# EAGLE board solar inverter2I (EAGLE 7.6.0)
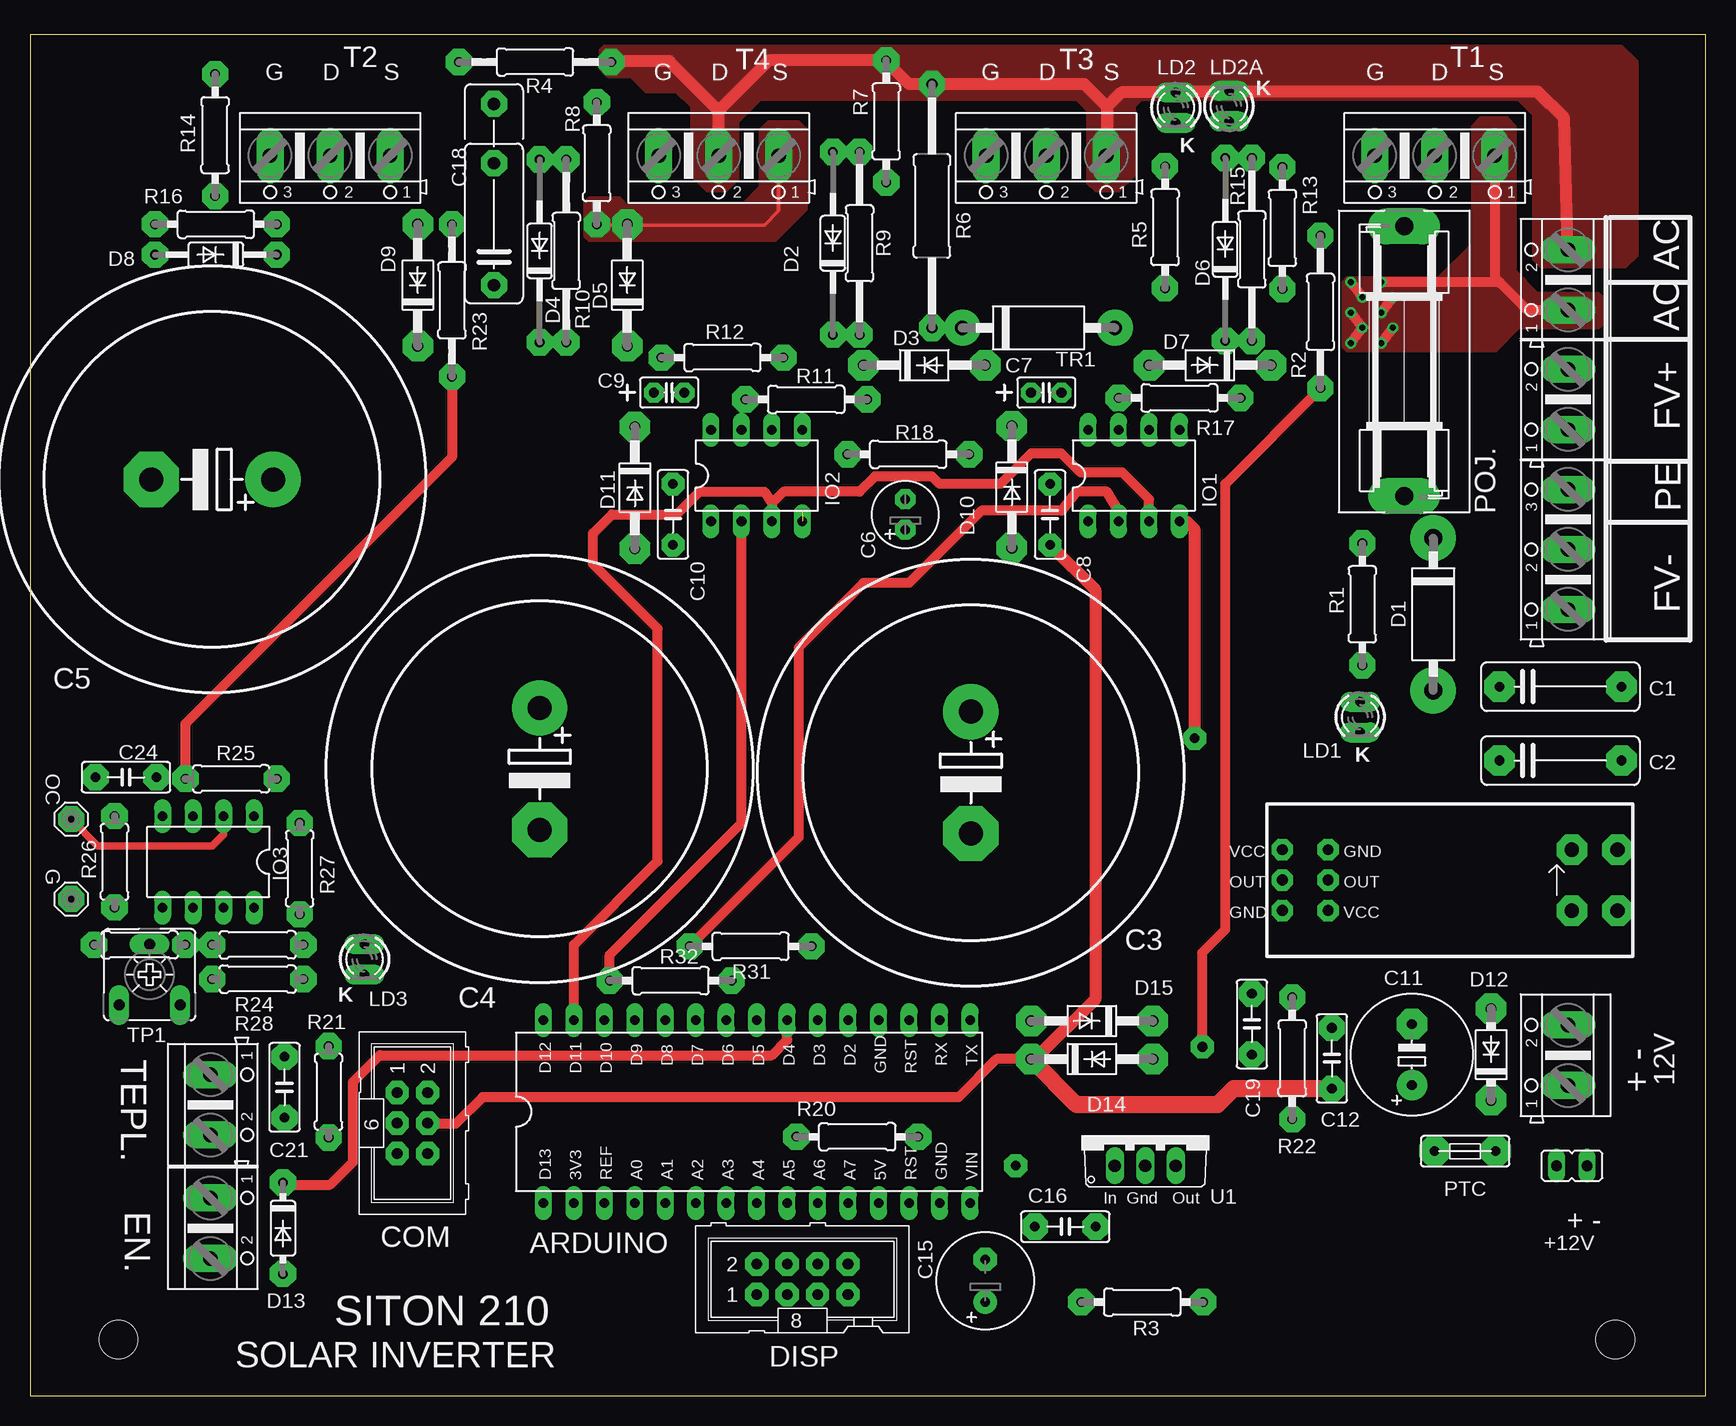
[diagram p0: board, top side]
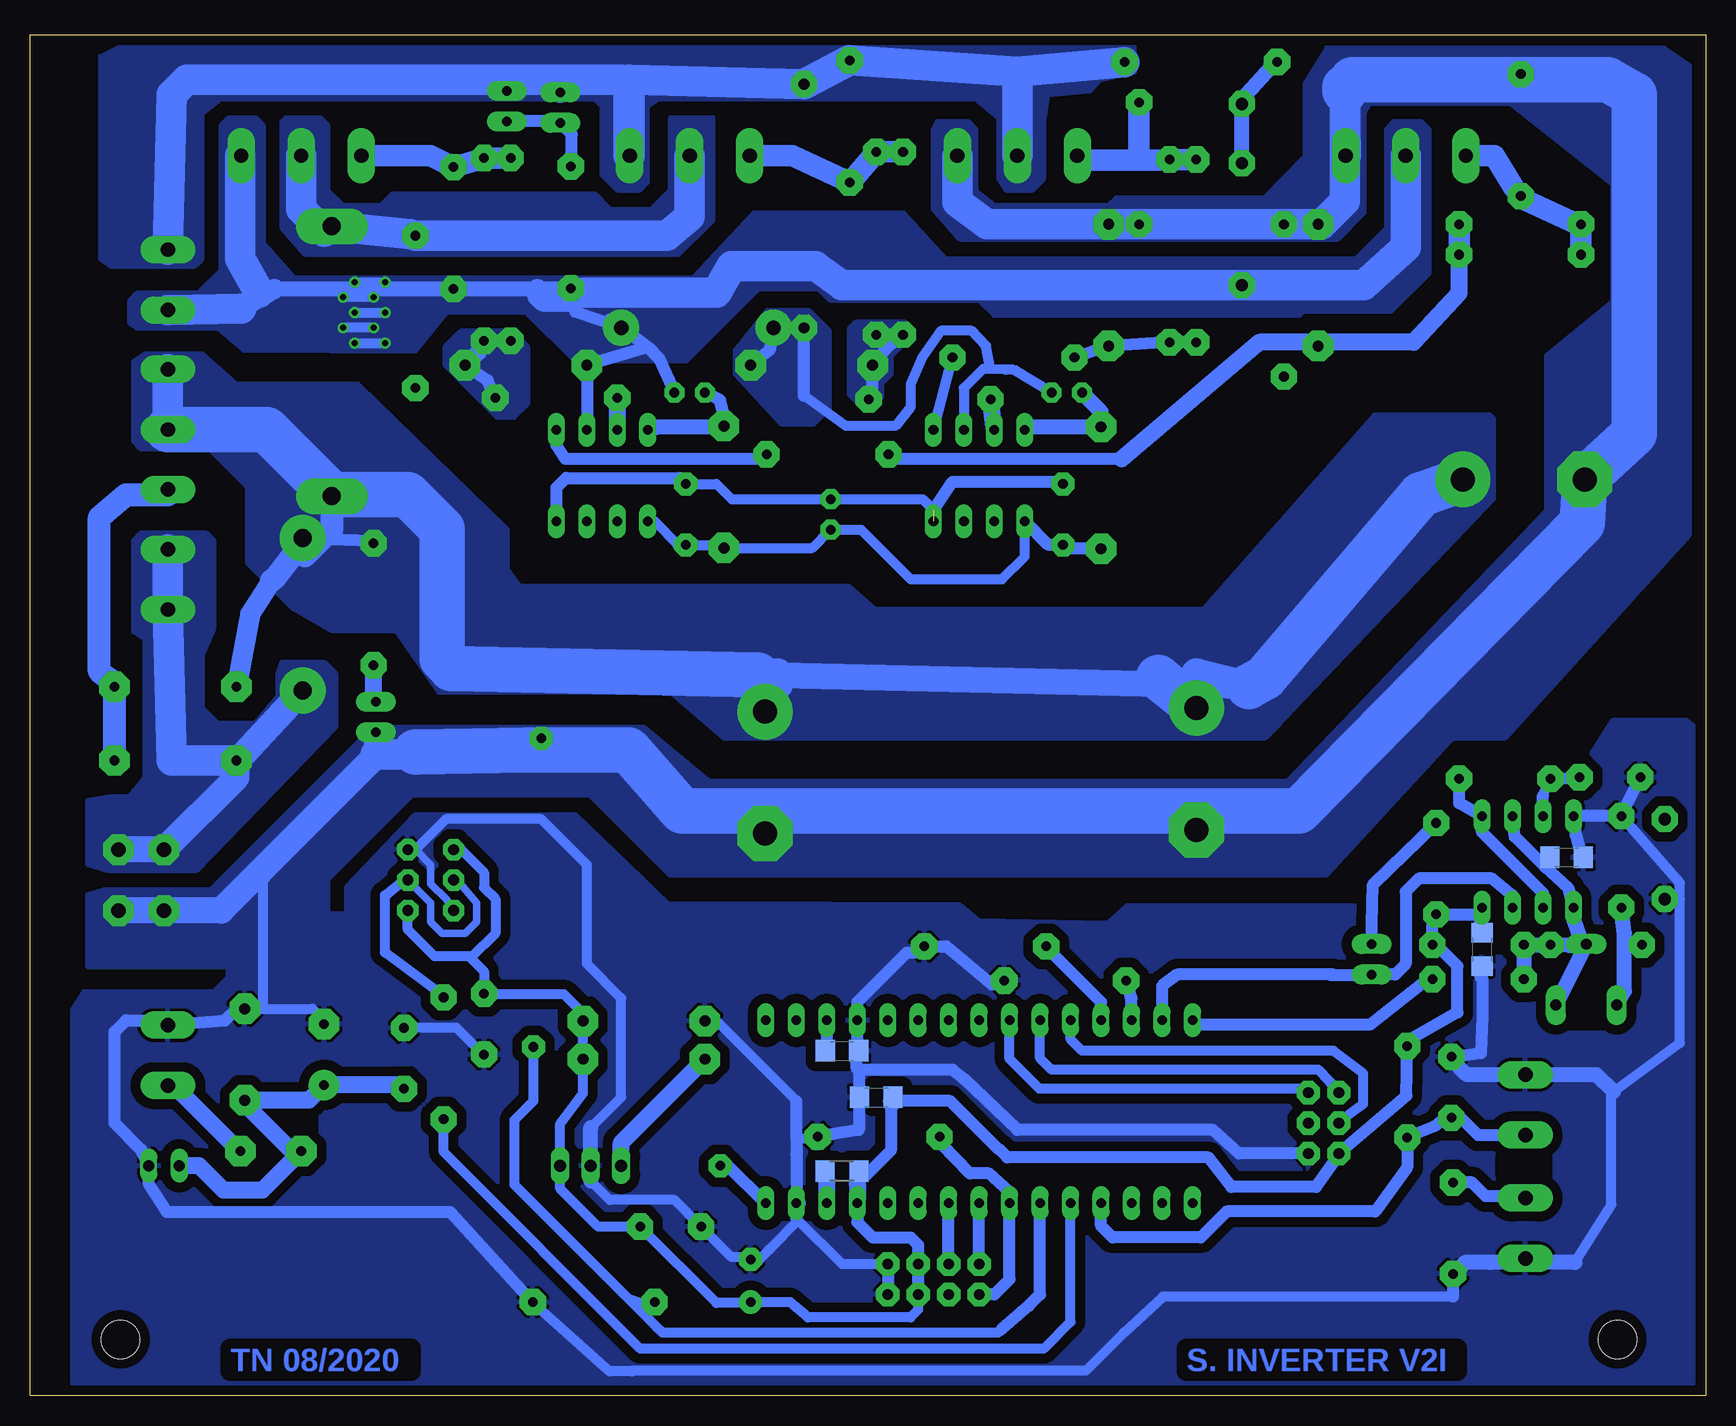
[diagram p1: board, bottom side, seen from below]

Size 139.7 x 113.47 mm. Coordinates in mm from the lower left corner, seen from the top.
Outline: 139.7,113.47 0,113.47 0,0 139.7,0 139.7,113.47
Copper layers (1*16): Top 0.035mm / dielectric 1.5mm / Bottom 0.035mm
Design rules "default *": minimum track width 10mil, minimum drill 24mil, track to track 8mil, track to pad 8mil, pad to pad 8mil, via to via 8mil, smd to smd 8mil, copper to edge 15mil, drill to drill 8mil, minimum pad ring 10mil, minimum via ring 8mil, stop-mask expansion 4mil, vias tented up to drill 0mil, thermal gap 10mil
Holes 3.2 mm at 132.14,4.7 7.37,4.7
bRestrict: area 71.6,27.9 to 72.3,30.2; area 68.9,24.1 to 69.5,25.8; area 74.3,15.4 to 77,16.5; area 7.6,31.2 to 12.3,37.3; area 13.6,18.5 to 16.8,19.8; area 116.5,22 to 118.4,23.6

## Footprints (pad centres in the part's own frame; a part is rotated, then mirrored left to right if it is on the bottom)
AK500/2 = drill 1.2 pad 2.311 long: 1 -2.515,0; 2 2.515,0
JP1 = drill 0.9 pad 1.422 long: 1 0,-1.27; 2 0,1.27
DIL30 = drill 0.8 pad 1.422 long: 1 -16.51,-7.62; 2 -13.97,-7.62; 3 -11.43,-7.62; 4 -8.89,-7.62; 5 -6.35,-7.62; 6 -3.81,-7.62; 7 -1.27,-7.62; 8 1.27,-7.62; 9 3.81,-7.62; 10 6.35,-7.62; 11 8.89,-7.62; 12 11.43,-7.62; 13 13.97,-7.62; 14 16.51,-7.62; 15 19.05,-7.62; 18 19.05,7.62; 19 16.51,7.62; 20 13.97,7.62; 21 11.43,7.62; 22 8.89,7.62; 23 6.35,7.62; 24 3.81,7.62; 25 1.27,7.62; 26 -1.27,7.62; 27 -3.81,7.62; 28 -6.35,7.62; 29 -8.89,7.62; 30 -11.43,7.62; 31 -13.97,7.62; 32 -16.51,7.62
C10B4 = drill 0.8 pad 2.54 octagon: 1 -5.08,0; 2 5.08,0
EB35D = drill 2 pad 4.597: + -5.08,0 | drill 2 pad 4.597 octagon: - 5.08,0
E2,5-6 = drill 0.8 pad 1.676 octagon: + -1.27,0; - 1.27,0
C025-025X050+ = drill 0.8 pad 1.676 octagon: 1 -1.27,0; 2 1.27,0
C050-025X075 = drill 0.8 pad 1.93 octagon: 1 -2.54,0; 2 2.54,0
E5-10,5 = drill 0.8 pad 2.54: + -2.54,0 | drill 0.8 pad 2.54 octagon: - 2.54,0
C050-025X075' = drill 0.8 pad 2.184 octagon: 1 -2.54,0; 2 2.54,0
C1206 = smd 1.6 x 1.8: 1 -1.4,0; 2 1.4,0
E3,5-8 = drill 0.8 pad 1.93: + -1.778,0 | drill 0.8 pad 1.93 octagon: - 1.778,0
C10-15B6 = drill 1.016 pad 2.159 octagon: 1 -5.08,0; 2 5.08,0; 3 10.033,0
ML6 = drill 0.9 pad 1.93 octagon: 1 -2.54,-1.27; 2 -2.54,1.27; 3 0,-1.27; 4 0,1.27; 5 2.54,-1.27; 6 2.54,1.27
DO15-12-1.5 = drill 1.5 pad 3.81: A 6.35,0; C -6.35,0
DO35-15 = drill 0.8 pad 2.184 octagon: A 7.62,0; C -7.62,0
DO41-10 = drill 0.9 pad 2.54 octagon: A 5.08,0; C -5.08,0
DO35-10 = drill 0.8 pad 2.184 octagon: A 5.08,0; C -5.08,0
DO41-7 = drill 0.9 pad 2.54 octagon: A 3.81,0; C -3.81,0
DO35-7 = drill 0.8 pad 2.184 octagon: A 3.81,0; C -3.81,0
ML8 = drill 0.9 pad 1.93 octagon: 1 -5.08,-1.27; 2 -5.08,1.27; 3 -2.54,-1.27; 4 -2.54,1.27; 5 0,-1.27; 6 0,1.27; 7 2.54,-1.27; 8 2.54,1.27
ACS712V2 = drill 0.9 pad 1.778 octagon: P$1 3.81,5.08; P$2 0,0; P$3 0,2.54; P$4 0,5.08; P$5 3.81,2.54; P$7 3.81,0 | drill 1.2 pad 2.54 octagon: P$6 24.13,0; P$8 24.13,5.08; P$9 27.94,5.08; P$10 27.94,0
AK500/3 = drill 1.2 pad 2.311 long: 1 -5.004,0; 2 0,0; 3 5.004,0
MCS10B = drill 1.016 pad 2.159 octagon: MP 0,0
DIL08 = drill 0.8 pad 1.422 long: 1 -3.81,-3.81; 2 -1.27,-3.81; 3 1.27,-3.81; 4 3.81,-3.81; 5 3.81,3.81; 6 1.27,3.81; 7 -1.27,3.81; 8 -3.81,3.81
LED3MM = drill 0.8 pad 1.676 long: A -1.27,0; K 1.27,0
POJISTKA = drill 1.5 pad 3 long: 1 -11.252,0; 2 11.252,0
PTC_FUSE = drill 0.8 pad 2.54 octagon: 1 -2.54,0; 2 2.54,0
0207/10 = drill 0.8 pad 2.184 octagon: 1 -5.08,0; 2 5.08,0
0207/12 = drill 0.8 pad 2.184 octagon: 1 -6.35,0; 2 6.35,0
0309/20 = drill 0.9 pad 2.184 octagon: 1 -10.16,0; 2 10.16,0
0207/15 = drill 0.8 pad 2.184 octagon: 1 -7.62,0; 2 7.62,0
R1206 = smd 1.6 x 1.803: 1 -1.422,0; 2 1.422,0
0207/7 = drill 0.8 pad 2.184 octagon: 1 -3.81,0; 2 3.81,0
CA6V = drill 0.9 pad 1.676 long: A -2.54,-2.54; E 2.54,-2.54; S 0,2.54
DO15-12 = drill 1.2 pad 3: A 6.35,0; C -6.35,0
TO220V = drill 1.016 long: 1 -2.54,-2.54; 2 0,-2.54; 3 2.54,-2.54

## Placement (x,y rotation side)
12V  + 12V -  [AK500/2]  128.21,28.38 90 top
+12V  +12V-  [JP1]  128.52,19.18 90 top
ARDUINO  Arduino Nano  [DIL30]  59.31,23.69 0 top
C1  100n/275V  [C10B4]  127.57,59.12 0 top
C2  100n/275V  [C10B4]  127.57,52.96 0 top
C3  470u/450V  [EB35D]  78.42,51.94 270 top
C4  470u/450V  [EB35D]  42.48,52.26 270 top
C5  470u/450V  [EB35D]  15.18,76.39 180 top
C6  10u  [E2,5-6]  72.96,73.47 90 top
C7  10u  [C025-025X050+]  84.71,83.63 0 top
C8  100n  [C050-025X075]  85.03,73.47 270 top
C9  10u  [C025-025X050+]  53.28,83.63 0 top
C10  100n  [C050-025X075]  53.59,73.47 270 top
C11  470uF  [E5-10,5]  115.19,28.45 90 top
C12  100n  [C050-025X075']  108.52,28.13 90 top
C13  100n  [C1206]  69.15,24.89 0 bottom
C14  100n  [C1206]  72.01,28.77 0 bottom
C15  220uF  [E3,5-8]  79.63,9.59 90 top
C16  100n  [C050-025X075']  86.3,14.1 0 top
C18  15n  [C10-15B6]  38.67,97.66 90 top
C19  100n  [C050-025X075']  101.85,30.99 90 top
C21  100n  [C050-025X075']  21.21,25.72 270 top
C24  33n  [C050-025X075']  8,51.56 180 top
C25  100n  [C1206]  11.62,44.89 0 bottom
C26  100n  [C1206]  18.67,37.21 270 bottom
COM  [ML6]  31.88,22.73 270 top
D1  15A10G  [DO15-12-1.5]  116.97,65.15 270 top
D2  1N4148  [DO35-15]  66.93,96.08 90 top
D3  P6KE18A  [DO41-10]  74.55,85.92 0 top
D4  1N4148  [DO35-15]  42.48,95.44 90 top
D5  P6KE18A  [DO41-10]  49.78,92.58 90 top
D6  1N4148  [DO35-15]  99.63,95.57 90 top
D7  P6KE18A  [DO41-10]  98.36,85.92 180 top
D8  1N4148  [DO35-10]  15.49,95.12 180 top
D9  P6KE18A  [DO41-10]  32.32,92.58 90 top
D10  UF4007  [DO41-10]  81.85,75.76 270 top
D11  UF4007  [DO41-10]  50.42,75.69 270 top
D12  P6KE15A  [DO41-7]  121.79,28.45 90 top
D13  ZD5V1  [DO35-7]  21.08,13.97 270 top
D14  1N4007  [DO41-10]  88.52,28.07 0 top
D15  ZD5V6  [DO41-10]  88.52,31.24 180 top
DISP  [ML8]  65.66,9.72 0 top
E$2  [ACS712V2]  104.39,40.45 0 top
E$11  [AK500/3]  128.21,70.55 90 top
E$13  [AK500/2]  128.21,83.06 90 top
E$14  [AK500/2]  128.21,93.03 90 top
EN.  EN.  [AK500/2]  15.05,13.97 270 top
G  [MCS10B]  3.43,41.4 0 top
IO1  IR2104  [DIL08]  92.01,76.71 0 top
IO2  IR2104  [DIL08]  60.58,76.71 0 top
IO3  [DIL08]  14.86,44.51 180 top
LD1  [LED3MM]  110.87,56.58 270 top
LD2  [LED3MM]  95.5,107.38 270 top
LD2A  [LED3MM]  99.95,107.51 90 top
LD3  [LED3MM]  27.88,36.39 270 top
OC  [MCS10B]  3.43,48.07 0 top
POJ.  [POJISTKA]  114.55,86.23 90 top
PTC  400mA  [PTC_FUSE]  119.63,20.38 180 top
R1  300k  [0207/10]  111.06,65.98 90 top
R2  470K  [0207/12]  107.57,90.36 90 top
R3  5k6  [0207/10]  92.71,7.81 180 top
R4  10R  [0207/12]  42.1,111.19 0 top
R5  300k  [0207/10]  94.61,97.41 90 top
R6  0R1  [0309/20]  75.18,99.19 90 top
R7  22k  [0207/10]  71.37,106.24 90 top
R8  22k  [0207/10]  47.24,102.74 90 top
R9  100R  [0207/15]  69.15,96.08 90 top
R10  100R  [0207/15]  44.7,95.44 90 top
R11  10R  [0207/10]  64.71,83.06 180 top
R12  10R  [0207/10]  57.72,86.55 0 top
R13  22k  [0207/10]  104.39,97.35 90 top
R14  22k  [0207/10]  15.43,105.09 270 top
R15  100R  [0207/15]  101.85,95.57 90 top
R16  100R  [0207/10]  15.49,97.66 0 top
R17  10R  [0207/10]  95.82,83.19 180 top
R18  10R  [0207/10]  73.22,78.49 0 top
R19  1k  [R1206]  72.01,18.73 0 bottom
R20  10k  [0207/10]  68.96,21.59 0 top
R21  2k2  [0207/7]  24.89,25.34 90 top
R22  560  [0207/10]  105.22,28.13 90 top
R23  10k  [0207/12]  35.18,91.31 90 top
R24  100k  [0207/7]  18.99,37.59 0 top
R25  33k  [0207/7]  16.76,51.44 0 top
R26  1k5  [0207/7]  7.05,44.51 90 top
R27  1k  [0207/7]  22.48,43.94 90 top
R28  560  [0207/7]  18.99,34.73 0 top
R31  10k  [0207/10]  60.07,37.47 0 top
R32  10k  [0207/10]  53.4,34.61 0 top
T1  47N60  [AK500/3]  117.09,103.38 180 top
T2  47N60  [AK500/3]  25.02,103.38 180 top
T3  47N60  [AK500/3]  84.71,103.38 180 top
T4  47N60  [AK500/3]  57.4,103.38 180 top
TEPL.  TEPL.  [AK500/2]  15.05,24.26 270 top
TP1  5k  [CA6V]  9.97,35.12 0 top
TP2  [0207/7]  9.14,37.59 180 top
TR1  1,5KE440CA  [DO15-12]  84.07,89.03 0 top
U1  LM7805  [TO220V]  92.96,21.72 0 top

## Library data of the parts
12V +12V ARDUINO C1-C6 C12-C14 C16 C18 C19 C21 C24-C26 COM D1-D15 DISP E$2 E$11 E$13 E$14 EN. IO1-IO3 POJ. PTC R1-R28 R31 R32 T1-T4 TEPL. TP1 TP2 TR1 = 11moje
C7-C11 C15 = 12moje
G OC = solpad
LD1 LD2 LD2A LD3 = 10moje
U1 = linear

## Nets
+5V: ARDUINO.12 C13.2 C15.+ C16.2 C19.2 C26.1 COM.5 D14.A D15.C DISP.5 DISP.6 E$2.P$4 E$2.P$7 IO3.8 R19.2 R21.2 R24.2 R27.1 U1.3
+12V: +12V.2 C6.+ C8.2 C10.2 C11.+ C12.1 COM.4 D10.A D11.A D12.C D14.C IO1.1 IO2.1 PTC.2 U1.1
AC1: E$14.2 LD2.A LD2A.K R4.2 R6.2 R7.2 T3.1 T4.2
AC2: C7.2 C18.1 D7.A E$14.1 IO1.6 R5.1 R13.1 T1.1 T2.2 TR1.A
MINUS-FP: C2.1 D1.A E$2.P$8 E$2.P$9 E$11.1 E$11.2
MINUS-GND: 12V.2 +12V.1 ARDUINO.14 ARDUINO.21 C3.- C4.- C5.- C6.- C8.1 C10.1 C11.- C12.2 C13.1 C14.2 C15.- C16.1 C19.1 C21.1 C24.2 C25.2 C26.2 COM.6 D5.A D9.A D12.A D13.A D15.A DISP.7 DISP.8 E$2.P$1 E$2.P$2 E$2.P$6 E$2.P$10 EN..2 G.MP IO1.4 IO2.4 IO3.4 LD1.K R3.1 R8.1 R14.1 R20.2 R23.2 R26.2 R31.2 R32.2 T2.1 T4.1 TEPL..1 U1.2
PLUS: POJ..2 R2.2 T1.2 T3.2
PLUS-FP: C1.1 C3.+ C4.+ C5.+ D1.C E$13.1 E$13.2 POJ..1 R1.2
S$1: IO1.7 R17.2
S$2: ARDUINO.5 R22.1
S$3: IO3.1 IO3.6 R25.2
S$4: D6.C D7.C R15.1 R17.1
S$5: ARDUINO.30 IO2.2 R32.1
S$6: ARDUINO.7 DISP.1 R20.1
S$7: C1.2 C2.2 E$11.3
S$8: LD2.K LD2A.A R5.2
S$9: ARDUINO.13 R19.1
S$10: C9.1 D11.C IO2.8
S$11: D8.A R14.2 R16.1 T2.3
S$12: D8.C D9.C R16.2 R18.1
S$13: IO1.5 R18.2
S$14: C7.1 D10.C IO1.8
S$15: ARDUINO.29 IO1.2 R31.1
S$16: IO2.7 R11.2
S$17: LD1.A R1.1
S$18: D2.A R7.1 R9.2 T3.3
S$19: D2.C D3.C R9.1 R11.1
S$20: D4.A R8.2 R10.2 T4.3
S$21: D4.C D5.C R10.1 R12.1
S$22: IO2.5 R12.2
S$23: ARDUINO.20 C14.1
S$24: D6.A R13.2 R15.2 T1.3
S$25: ARDUINO.15
S$26: ARDUINO.28 COM.3
S$27: C18.2 R4.1
S$28: ARDUINO.27 COM.1
S$29: C9.2 D3.A IO2.6 R6.1 TR1.C
S$30: ARDUINO.26 COM.2
S$31: ARDUINO.8 DISP.2
S$32: ARDUINO.9 DISP.4
S$33: ARDUINO.4 C21.2 R21.1 TEPL..2
S$34: C24.1 IO3.3 R23.1 R25.1
S$36: ARDUINO.23
S$37: C25.1 IO3.2 IO3.5 OC.MP R24.1 R28.1 TP1.E TP1.S TP2.1
S$38: R26.1 TP1.A TP2.2
S$39: ARDUINO.24 D13.C EN..1
S$40: LD3.A R27.2
S$41: ARDUINO.6 R2.1 R3.2
S$42: ARDUINO.22
S$43: ARDUINO.31 IO1.3 IO2.3 IO3.7 LD3.K
S$44: ARDUINO.32 R28.2
S$45: 12V.1 PTC.1
S$51: E$2.P$3 E$2.P$5 R22.2

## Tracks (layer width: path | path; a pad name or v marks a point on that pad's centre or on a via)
+5V
  Bottom 0.61: R19.2 70.59,18.45 70.74,17.65 | C13.2 67.88,23.68
  Bottom 0.813: DISP.5 65.66,7.17 66.29,6.54 74.87,6.54 76.33,7.81 C15.+ 79.38,7.81 79.31,7.75 82.49,7.75 C16.2 92.33,14.1 95.5,17.27 U1.3 95.5,22.67 93.6,25.21 D14.A D15.C 93.6,31.88 95.19,33.46 101.79,33.46 C19.2 | E$2.P$7 108.2,38.86 105.98,36.64 103.12,36.64 102.97,36.48 | 102.97,36.48 101.85,35.37 C19.2 | C19.2 101.85,33.46 | E$2.P$4 103.76,45.53 101.85,43.62 101.85,42.35 100.9,41.4 100.9,38.54 102.97,36.48 | 102.97,36.48
  Bottom 1.016: DISP.5 DISP.6 65.66,12.57 66.29,13.21 69.47,13.21 70.74,14.48 ARDUINO.12 70.74,16.38 | 70.59,18.45 69.94,18.45 67.94,20.45 67.94,24.07 67.75,24.26 C13.2 67.75,24.19 68.14,24.57 62.99,24.57 58.93,20.51 58.86,20.51 58.23,19.88 41.47,19.88 39.56,17.4 32.51,17.4 31.18,19.3 COM.5 24.96,25.02 R21.2 24.7,29.65 20.7,31.94 20.7,35.81 22.42,37.53 22.73,37.59 R24.2 | C26.1 18.86,38.99 18.8,38.29 18.67,38.54 IO3.8 18.8,39.43 18.73,40.13 R27.1 | R27.1 22.42,39.62 | R27.1 22.8,39.24 R24.2 | R24.2 22.8,37.53
  Bottom 1.422: 70.74,17.65 70.74,16.38
+12V
  Top 0.813: D14.C 80.58,28.07 77.41,24.89 37.72,24.89 35.5,22.67 33.21,22.67 COM.4
  Top 1.016: D14.C 83.76,28.07 88.84,33.15 88.84,67.12 C8.2
  Top 1.422: C12.1 100.33,25.59 99,24.26 87.25,24.26 D14.C
  Bottom 0.813: IO1.1 87.63,72.9 85.66,70.93 | C8.2 82.11,70.93 | IO2.1 56.77,69.98 58.67,68.07 66.29,68.07 70.42,72.2 C6.+ 74.49,70.68 D10.A
  Bottom 1.016: 85.66,70.93 C8.2 | 82.11,70.93 D10.A | D11.A 53.28,70.61 C10.2 54.8,70.93 IO2.1
  Bottom 1.422: +12V.2 125.6,19.18 123.57,17.14 120.33,17.14 PTC.2 117.86,20.38 122.17,24.7 | 122.17,24.7 122.24,24.77 | 122.17,24.7 D12.C 116.46,24.64 C11.+ 108.84,25.91 C12.1 | U1.1 90.42,21.08 D14.C
AC1
  Top 0.305: T3.1 89.71,107.52 | T4.2 57.4,103.31
  Top 1.016: E$14.2 127.89,106.49 125.67,108.71 95.5,108.71 | LD2.A 91,108.65 89.79,107.44 89.79,103.31 | 89.71,107.52 87.88,109.35 R6.2 73.28,109.35 71.37,111.25 | R7.2 61.59,111.32 57.4,107.12 | T4.2 57.4,107.12 | 57.4,107.12 53.28,111.25 48.51,111.25
  Bottom 0.813: 89.79,109.73 90.42,109.73
  Bottom 1.016: 99.31,109.73 LD2A.K
  Bottom 1.676: E$14.2 127.89,95.76
  Bottom 1.778: 96.46,109.98 94.87,109.73 LD2.A
  Bottom 2.54: E$14.2 127.89,108.46 126.62,109.73 99.31,109.73 94.87,109.73 90.42,109.73 | 89.79,109.73 89.79,103.38 T3.1 89.71,109.73 R6.2 R7.2 57.4,110.36 | 57.4,110.36 T4.2 | R4.2 57.4,110.36
  pour Bottom (no thermals): 58.36,100.52 56.13,100.52 55.18,101.47 55.18,106.24 54.86,108.46 51.31,108.78 50.48,109.73 47.62,110.36 47.62,112.39 132.33,112.39 133.86,111.63 133.86,94.81 132.97,94.17 125.98,94.17 125.35,94.81 125.35,106.87 123.76,108.14 92.65,108.14 92.01,107.51 92.01,101.79 90.74,100.52 88.84,100.52 88.2,101.16 88.2,107.51 87.25,108.14 60.9,108.14 58.99,106.55 58.99,101.47
  pour Top (no thermals): 125.98,94.11 132.97,94.11 133.92,95.06 133.92,111.25 132.65,112.52 47.88,112.52 47.56,112.2 47.56,110.62 48.2,109.98 50.1,109.98 51.37,108.71 53.91,108.71 55.18,107.44 55.18,101.73 56.45,100.46 58.04,100.46 58.99,101.41 58.99,106.17 60.9,108.08 87.25,108.08 88.2,107.12 88.2,101.09 88.84,100.46 90.74,100.46 92.01,101.73 92.01,107.44 92.65,108.08 124.08,108.08 125.35,106.81 125.35,94.74
AC2  (via drill 0.5)
  Top 0.813: E$14.1 124.82,90.51 122.49,92.84 122.17,92.84 | 122.17,92.84 v112.65,92.84 | v110.11,92.84 v111.06,91.57 | v113.6,91.57 v112.65,90.3 | v110.11,90.3 v111.06,89.03 v110.11,87.76 | v113.6,89.03 v112.65,87.76 | T1.1 122.1,92.91 122.17,92.84
  Bottom 0.813: v112.65,92.84 v110.11,92.84 | v111.06,91.57 v113.6,91.57 | v112.65,90.3 v110.11,90.3 | v111.06,89.03 v113.6,89.03 | v112.65,87.76 v110.11,87.76
  Bottom 1.016: IO1.6 D7.A 88.2,87.41 | 94.23,91.63 94.23,90.36 90.3,89.03 | 90.3,89.03 91.38,89.73 TR1.A 90.3,89.03 | 90.3,89.03 88.2,87.41 | 87.25,86.46 88.2,87.44 | 88.2,87.41 87.25,86.46 | 87.25,86.46 C7.2
  Bottom 1.27: 97.41,92.27 R13.1 119.32,92.27
  Bottom 1.676: R5.1 94.23,91.63 | 93.6,91.95 94.23,92.27 R5.1 | 97.41,91.63 96.77,91.63 97.41,92.27 | 120.59,91.95 119.32,92.27 122.11,90.61 | 122.17,103.38 T1.1 | 94.55,91.63 94.55,91.95 R5.1 | 36.45,92.58 36.13,92.27
  Bottom 2.54: T2.2 25.02,95.76 28.51,92.58 36.45,92.58 C18.1 72.01,92.58 74.23,94.17 81.22,94.17 82.49,91.95 93.6,91.95 | 120.59,91.95 122.17,94.8 122.17,103.38 | 122.11,90.61 E$14.1 | 94.55,91.63 96.77,91.63
  pour Bottom (no thermals): 130.75,91.95 125.67,91.95 123.76,93.85 123.76,105.92 123.13,106.55 120.9,106.55 120.27,105.92 120.27,96.08 117.73,93.22 84.39,93.22 79.31,98.62 66.93,98.62 63.44,94.81 29.15,94.81 26.61,97.35 26.61,105.6 25.97,106.24 23.75,106.24 23.11,105.6 23.11,93.54 26.29,90.36 33.59,90.36 33.91,90.04 59.31,90.04 60.58,91.31 72.96,91.31 73.91,92.27 78.99,92.27 85.03,86.23 94.23,86.23 98.3,90.3 105.03,90.3 107.63,87.06 121.86,87.12 124.02,88.96 130.75,88.96 131.38,89.41 131.38,91.31
  pour Top (no thermals): 130.75,91.88 125.67,91.88 123.76,93.79 123.76,105.85 123.13,106.49 120.9,106.49 120.27,105.85 120.27,96.01 117.41,93.15 109.79,93.15 109.47,92.84 109.47,87.44 109.79,87.12 122.17,87.12 124.08,89.03 130.75,89.03 131.06,89.34 131.06,91.57
MINUS-FP
  Bottom 2.184: D1.A 121.86,53.53 C2.1 122.49,51.56 E$2.P$8 E$2.P$9
  Bottom 2.54: E$11.2 E$11.1 127.89,52.96 C2.1
  pour Bottom (no thermals): 130.43,71.95 125.03,71.95 124.4,71.31 124.4,64.01 125.35,61.79 125.35,57.34 124.08,56.07 120.9,56.07 119,58.29 119,60.2 118.68,61.15 115.19,61.15 114.24,60.2 114.24,55.75 125.86,43.75 133.16,43.75 134.87,44.26 134.87,49.66 132.97,49.97 131.38,49.97 130.11,51.56 130.11,63.06 131.06,63.69 131.06,71.31
MINUS-GND  (via drill 0.8 pad 1.93)  (1 unrouted)
  Top 0.305: T4.1 62.41,98.79 61.21,97.6 47.56,97.6
  Top 1.016: v97.09,54.8 97.09,72.2 96.39,72.9 IO1.4
  Bottom 0.406: G.MP 2.16,41.4
  Bottom 0.61: 70.74,24 70.61,24.77 C13.1 70.61,24.45 | 75.82,18.92 75.69,19.05 75.69,18.73 | E$2.P$2 105.03,41.4 106.3,42.67 106.3,44.26 107.57,45.53 E$2.P$1
  Bottom 0.813: R23.2 31.69,97.98 32,97.66 | DISP.8 72.01,10.99 75.66,14.64 | 75.82,14.79 75.66,14.64 | 75.66,14.64 | 75.66,14.64 78.07,12.22 | 78.07,12.22 78.17,12.13 | C19.1 101.85,28.38 104.14,30.67 C12.2 | C11.- 115.19,31.3 116.14,32.26 120.27,32.26 | 120.59,43.62 120.27,43.31 120.27,32.26 | D12.A 120.27,32.26 | C21.1 21.34,28.19 | R26.2 2.16,42.73 2.16,41.4 2.16,29.4 7.72,25.35 7.84,25.25 7.87,25.25 7.87,15.94 10.92,11.11 | 21.08,8.26 45.28,8.26 48.51,5.27 51.69,2.09 89.47,2.09 89.47,2.03 91.38,2.03 R3.1 | EN..2 15.37,11.37 17.97,11.11 | D15.A 82.49,31.24 75.82,24.57 | 92.96,17.91 91.38,16.32 85.98,16.32 C16.1 81.22,11.56 79.95,11.56 79.63,11.24 C15.- 78.87,11.37 78.04,12.19 78.07,12.22 | 78.07,12.22 | 107.57,45.53 105.03,48.07 97.09,48.07 93.28,44.26 93.28,36 90.42,33.15 90.42,24.89 92.96,22.35 | 72.9,21.78 74.1,21.4 75.82,21.4 | 75.69,19.05 75.82,19.18 75.82,20.13 | C8.1 82.49,76.01 81.22,74.74 C6.- 65.28,74.74 64.39,73.85
  Bottom 1.016: R32.2 59.5,34.29 63.31,37.47 R31.2 65.66,36.96 66.61,36.96 70.74,32.83 ARDUINO.21 70.74,28.7 | COM.6 38.93,20.19 41.08,22.16 57.4,22.16 61.85,26.42 62.8,27.18 70.42,27.18 70.59,27.18 70.59,27.14 70.61,27.11 | C14.2 70.68,28.77 70.74,28.7 | 70.74,28.7 70.8,28.64 70.8,27.3 70.61,27.11 | C13.1 70.55,24.32 70.61,24.26 | 70.61,27.11 70.61,24.26 | 70.61,24.26 70.61,22.16 72.9,21.78 R20.2 | 75.82,15.94 75.76,15.88 | 75.82,15.94 75.95,16.07 | DISP.8 DISP.7 | 75.82,15.94 75.82,14.79 | 75.82,15.94 ARDUINO.14 75.82,20.13 75.82,21.4 75.82,24.57 | 14.54,109.73 15.18,109.09 | 64.39,73.85 62.8,76.2 53.59,76.2 C10.1 | IO1.4 95.82,75.69 95,76.52 85.53,76.52 C8.1 | v97.09,54.8 98.36,54.16 98.36,53.85 | 110.87,53.47 LD1.K | D12.A 122.49,32.26 123.47,31.28 12V.2 128.21,31.3 131.7,31.3 132.65,30.35 132.65,22.73 130.43,20.51 +12V.1 129.79,17.65 128.27,15.3 104.65,15.3 R3.1 | 18.79,34.86 18.8,34.86 | 18.79,34.86 C26.2 | 18.79,34.86 18.61,34.67 18.61,31.62 18.73,28.57 C21.1 | C25.2 10.41,45.15 10.86,46.74 IO3.4 R26.2 C24.2 | D13.A 21.08,8.26
  Bottom 1.27: C5.- 10.1,76.33 | C21.1 21.21,28.07 19.91,26.77 TEPL..1 9.12,26.77 7.72,25.37 7.72,25.35 | D13.A 21.02,10.16 20.07,11.11 17.97,11.11 10.92,11.11 | 92.96,17.91 U1.2 92.96,22.35
  Bottom 1.422: ARDUINO.14 75.76,16.07 | LD1.K 110.87,54.86 110.74,54.74
  Bottom 1.676: 14.22,109.73 R14.1
  Bottom 2.184: E$2.P$10 E$2.P$6 123.76,40.45 120.59,43.62 110.74,53.47 110.74,54.74
  Bottom 2.54: T4.1 62.41,99.49 59.94,97.66 R8.1 | R8.1 45.34,97.66 | R8.1 32,97.66 30.1,99.57 30.1,108.77 T2.1 | 29.46,109.73 30.1,109.09 | 14.22,109.73 14.54,109.73 | 8.35,109.57 8.19,109.41 | 8.35,109.57 8.51,109.73 | 8.35,109.57 | 8.19,109.73 8.35,109.57 | C5.- 9.78,76.71 | 107.39,53.66 107.38,53.66 107.38,53.47 | 107.38,53.47 107.38,53.34 | 107.38,53.47 110.74,53.47 110.87,53.47
  Bottom 3.81: 30.1,109.09 30.1,108.77 | 14.54,109.73 29.46,109.73 | 8.51,109.73 14.22,109.73 | 8.19,109.73 5.97,108.46 5.97,80.2 9.78,76.71 | C5.- 10.29,72.77 33.91,48.77 42.16,48.77 | 77.72,48.77 C3.- | 42.16,48.77 C4.- | 77.72,48.77 42.16,48.77 | 77.72,48.77 85.34,48.77 89.79,53.85 98.36,53.85 107.39,53.66 107.57,53.66
  pour Bottom (no thermals): 61.21,104.97 63.75,104.97 63.75,100.2
  pour Bottom (no thermals): 133.48,42.23 124.59,42.23 111.06,55.75 88.52,55.75 83.12,51.31 34.86,51.24 13.27,73.79 13.27,86.74 7.75,91.25 7.75,100.96 16.32,107.7 28.07,107.7 28.51,106.87 28.51,98.62 30.73,96.39 62.17,96.39 64.39,98.93 64.39,105.6 64.07,106.24 61.53,106.24 60.9,105.6 60.9,100.52 59.31,99.25 49.78,99.25 49.15,99.89 36.77,99.89 33.4,103.31 33.4,109.41 31.56,112.39 3.49,112.39 1.4,110.93 1.4,71.75 16.76,54.8 21.15,54.8 21.53,54.42 31.69,43.37 86.3,43.37 92.96,50.04 107.89,50.04 114.87,43.05 114.87,40.2 117.09,35.75 134.87,35.75 134.87,41.78
  pour Bottom (isolate 0.813): 135.19,33.72 124.33,33.72 123.19,34.86 123.19,35.62 117.28,35.62 114.94,40.2 113.28,40.2 113.28,42.42 107.57,48.45 94.23,48.45 86.49,41.02 73.09,41.02 70.61,40.96 62.23,40.96 60.58,39.62 49.85,39.43 48.26,40.89 29.59,40.89 24.96,40.7 21.08,36.58 15.56,36.58 11.37,41.72 11.18,41.91 10.86,51.5 7.75,56.32 1.65,56.32 0.89,55.75 0.89,1.46 1.08,1.02 136.14,1.02 136.14,32.19
  pour Top (no thermals): 63.44,106.17 61.53,106.17 60.9,105.54 60.9,100.77 59.31,99.19 49.78,99.19 49.15,99.82 46.61,99.82 46.29,99.5 46.29,96.65 46.61,96.33 62.17,96.33 64.71,98.87 64.71,105.54 64.07,106.17
PLUS
  Bottom 2.54: T1.2 117.09,98.93 115.19,97.03 POJ..2 108.03,96.85 R2.2 86.61,96.71 84.71,98.3 T3.2
  pour Bottom (no thermals): 118.36,106.55 115.51,106.55 114.87,105.92 114.87,100.52 113.6,99.25 110.43,99.25 109.47,100.2 92.65,100.2 91.38,98.93 87.88,98.93 86.3,100.52 86.3,106.55 82.8,106.55 82.8,97.98 85.66,95.12 116.78,95.12 118.68,97.35 118.68,106.24
PLUS-FP
  Bottom 1.016: R1.2 111.19,71.06 111.19,71.31 D1.C
  Bottom 1.676: 119.57,67.94 121.35,65.15 C1.1
  Bottom 1.93: POJ..1 114.55,72.26 116.78,70.04 D1.C 117.09,70.99 119.32,68.13 119.57,67.94
  Bottom 2.184: 38.1,59.12 79.06,60.07
  Bottom 2.54: 114.55,75.12 POJ..1 | 79.06,60.07 77.41,59.88 | C3.+ 77.72,58.93 77.41,59.25 77.41,59.88 | 77.41,59.88 77.41,60.2 | 38.1,59.12 42.48,60.2 42.16,59.88 C4.+ | 127.89,80.2 E$13.1 E$13.2
  Bottom 3.81: E$13.1 119.98,80.54 114.55,75.12 108.2,75.12 105.35,72.26 105.35,61.47 104.58,60.64 79.06,60.07 | C5.+ 23.75,75.12 36.77,59.88 38.1,59.12 | C4.+ 45.66,59.88
  pour Bottom (no thermals): 130.11,86.87 125.35,86.87 122.49,84.33 112.33,84.33 99.95,72.26 99.95,68.9 98.87,67.5 71.44,67.5 69.28,65.6 41.85,65.6 27.56,81.79 18.03,81.79 17.72,81.47 17.72,74.8 36.77,54.8 81.85,54.8 86.3,58.61 105.6,58.61 109.16,63.69 114.55,63.75 117.73,65.6 121.54,69.41 121.54,75.76 124.71,78.93 130.43,78.93 131.06,79.57 131.06,86.23
S$1
  Bottom 1.016: R17.2 91.06,83.06
  Bottom 1.422: IO1.7 R17.2
S$2
  Bottom 0.813: R22.1 105.22,20.32 88.84,3.94 55.18,3.94 52.96,6.16 ARDUINO.5
S$3
  Bottom 0.813: IO3.6 13.59,40.77
  Bottom 1.016: R25.2 20.57,49.4 IO3.1 18.67,46.99 13.59,41.91 IO3.6
S$4
  Bottom 1.016: D6.C R15.1 D7.C | D7.C 102.17,86.87 | D7.C 101.54,84.65 R17.1
  pour Bottom (no thermals): 103.76,88.77 99.57,88.77 98.23,87.44 98.23,82.68 99.38,81.53 100.71,81.53 105.09,85.92 105.09,87.44
S$5
  Top 0.813: R32.1 48.32,36.77 59.31,47.75 IO2.2
  Bottom 1.016: R32.1 47.88,33.15 ARDUINO.30
S$6
  Bottom 1.016: DISP.1 59.31,8.45 58.04,9.71 ARDUINO.7 58.04,17.02 59.75,18.54 61.34,18.54 63.69,20.95 R20.1
S$7
  Bottom 1.93: C1.2 132.65,59.25 | C2.2 C1.2 | C1.2 132.65,59.44 133.92,60.39 133.92,73.21 131.7,75.12 128.21,75.12 127.89,75.44 E$11.3
S$8
  Bottom 1.016: R5.2 94.55,102.49 94.55,105.16 LD2.K 94.87,106.24 LD2A.A
S$9
  Bottom 1.016: 73.28,17.97 R19.1
  Bottom 1.422: ARDUINO.13 73.28,17.97
S$10
  Bottom 1.27: C9.1 50.42,82.04 D11.C 56.2,80.77 IO2.8
S$11
  Bottom 0.813: R16.1 10.73,97.66
  Bottom 1.778: T2.3 17.65,103.38 16,100.71 R14.2 15.49,99.88 10.73,97.66 | D8.A R16.1
S$12
  Bottom 0.813: 32.64,87.82 D9.C
  Bottom 1.016: 48.7,78.1 67.75,78.1 67.75,78.3 R18.1
  Bottom 1.422: 48.7,78.1 37.21,87.82 32.64,87.82 24.38,87.82 20.57,91.95 D8.C
  Bottom 1.778: D8.C R16.2
S$13
  Bottom 1.016: IO1.5 95.82,79.25 95.06,78.1 78.8,78.1 78.8,78.3 R18.2
S$14
  Bottom 1.016: D10.C 81.85,81.72 82.17,82.99 C7.1
  Bottom 1.27: 81.85,80.77 81.91,81.34 | D10.C 81.85,80.77 | IO1.8 87.31,80.77 81.85,80.77
S$15
  Top 0.813: IO1.2 90.74,73.79 89.79,75.38 87.25,75.38 85.98,73.79 79.31,73.79 73.28,67.75 69.47,67.75 64.07,62.36 64.07,46.55 R31.1
  Bottom 1.016: IO1.2 90.74,73.21 | ARDUINO.29 50.42,32.83 55.31,37.72 R31.1
S$16
  Bottom 1.422: IO2.7 R11.2
S$17
  Bottom 1.422: LD1.A 110.81,57.91 111.06,58.17 R1.1
S$18
  Bottom 1.778: T3.3 76.14,103.38 R7.1 71.06,101.47 R9.2 D2.A
S$19
  Bottom 1.016: R9.1 D2.C 68.2,87.5 D3.C 69.47,83.69 R11.1
  pour Bottom (no thermals): 69.66,82.3 70.23,82.3 71.37,83.44 71.37,88.96 70.8,89.53 66.8,89.53 66.55,88.65 66.55,88.07 67.94,86.68 67.94,85.15 68.71,84.39 68.71,83.25
S$20
  Bottom 1.778: D4.A R10.2 45.66,103 47.24,103 | T4.3 52.02,103 47.24,103 | 47.24,103 R8.2
S$21
  Bottom 1.016: R12.1 D5.C R10.1 D4.C
S$22
  Bottom 0.813: IO2.5 R12.2
S$23
  Bottom 1.016: C14.1 73.34,28.77 73.28,28.83 ARDUINO.20
S$24
  Bottom 1.778: T1.3 106.3,103.38 R13.2 R15.2 D6.A
S$25  (via drill 0.8 pad 1.93)
  Bottom 1.016: ARDUINO.15 78.36,16 81.53,19.18 v82.17,19.18
S$26
  Bottom 0.813: ARDUINO.28 52.96,29.72 52.01,28.77 31.05,28.77 28.58,26.86 28.58,24.32 30.73,22.73 COM.3
S$27
  Bottom 1.27: R4.1 35.81,111.25 38.67,108.08 C18.2
S$28
  Bottom 0.813: COM.1 31.37,26.23 32.32,27.18 54.55,27.18 55.5,28.13 ARDUINO.27
S$29
  Bottom 0.813: 75.18,83.38 71.69,80.84 67.56,80.84 66.29,82.42 66.29,84.33 65.34,86.55 63.75,88.77 61.21,88.77 60.01,87.5 59.63,85.6 | 59.63,85.6 60.26,85.6 61.85,84.01 IO2.6 | 59.63,85.6 58.36,85.53 57.72,85.53 C9.2
  Bottom 1.016: D3.A 78.04,87.19 TR1.C R6.1 75.18,83.38
  pour Bottom (no thermals): 80.9,85.15 80.9,87.19 78.23,90.49 74.8,90.49 73.09,88.77 73.09,82.3 74.42,80.96 77.03,80.96
S$30
  Bottom 0.813: ARDUINO.26 58.04,28.07 55.56,25.59 33.65,25.59 COM.2
S$31
  Bottom 1.016: DISP.2 ARDUINO.8
S$32
  Bottom 1.016: DISP.4 ARDUINO.9
S$33
  Bottom 1.016: ARDUINO.4 50.42,14.16 49.47,13.21 42.1,13.21 39.94,15.37 27.56,15.37 27.5,15.43 24.89,19.05 R21.1 22.61,22.48 21.46,23.43 C21.2 20.45,23.18 18.99,21.72 14.86,21.72 14.88,21.74 TEPL..2
S$34
  Top 0.813: R23.1 35.18,78.23 12.95,56.01 R25.1
  Bottom 0.813: 13.59,50.04 R25.1
  Bottom 1.016: IO3.3 13.59,50.04 | R25.1 C24.1
S$37
  Top 0.61: IO3.2 16.13,46.8 15.18,45.85 5.65,45.85 OC.MP
  Bottom 1.016: C25.1 13.59,44.45 13.4,44.07 | IO3.2 15.94,46.61 13.4,44.07 | 13.4,44.07 11.43,42.29 IO3.5 | TP1.S 10.22,38.1
  Bottom 1.27: TP1.S 10.41,38.1 10.99,39.62 IO3.5 | TP1.E TP1.S | TP1.S 11.37,37.53 R24.1 | R24.1 R28.1 | R24.1 TP2.1
S$38
  Bottom 1.27: R26.1 6.79,38.54 6.79,37.59 | 6.79,37.59 6.79,33.72 7.56,32.39 TP1.A | 6.79,37.59 TP2.2
S$39
  Top 0.813: 63.12,30.61 ARDUINO.24 63.12,29.65 61.85,28.38 29.15,28.38 26.92,26.16 26.92,19.49 25.02,17.59 21.27,17.59 D13.C
  Bottom 1.016: D13.C 19.49,17.78 18.35,16.64 15.18,16.64 15.02,16.48 | 15.02,16.48 14.86,16.32 | EN..1 15.02,16.48
S$40
  Bottom 0.813: R27.2 22.48,47.5
  Bottom 1.016: LD3.A 27.75,42.61 R27.2
S$41  (via drill 0.8 pad 1.93)
  Top 0.813: v97.73,29.08 97.73,36.96 99.63,38.86 99.63,76.01 107.57,83.95 R2.1
  Bottom 0.813: 86.93,5.27 58.99,5.27 58.67,5.59 | 86.93,5.27 86.99,5.27 | v97.73,29.08 97.73,24.57 99.31,22.99 99.31,17.59 89.79,8.06 | 86.93,5.27 87.57,5.84 89.79,8.06 | R3.2 88.58,7.68 89.79,8.06
  Bottom 1.016: ARDUINO.6 55.5,8.45 56.45,7.49 58.67,5.59
S$43
  Top 0.813: ARDUINO.31 45.34,37.59 52.32,44.58 52.32,63.95 46.93,69.34 46.93,71.88 48.51,73.47 53.91,73.47 55.82,75.38 61.21,75.38 61.85,74.42 | 61.85,74.42 IO2.3 | IO1.3 93.28,74.74 91.06,76.96 87.57,76.96 85.98,78.55 83.44,78.55 80.9,76.01 75.82,76.01 75.18,76.64 70.42,76.64 69.15,75.38 62.8,75.38 61.85,74.42
  Bottom 1.016: IO3.7 16.13,41.72 17.84,43.12 23.94,43.12 25.02,42.04 25.02,36 25.91,35.12 LD3.K 29.34,35.05 31.24,35.05 31.05,35.12 44.07,35.12 45.34,34.16 ARDUINO.31
S$44
  Bottom 1.016: ARDUINO.32 42.54,30.92 28,30.92 23.43,34.54 23.11,34.86 | 23.11,34.86 22.99,34.86 | R28.2 23.11,34.86
S$45
  Bottom 1.016: 127.25,25.27 128.21,26.23 12V.1
  Bottom 1.422: 12V.1 127.72,25.87 122.24,20.38 PTC.1
S$51
  Bottom 0.61: 104.08,42.99 102.49,41.09 102.49,39.5 103.44,38.54 105.35,38.54 106.3,39.5 106.3,41.09 E$2.P$5
  Bottom 0.813: R22.2 105.22,33.34 110.11,36.96 110.11,41.72 108.52,42.99 E$2.P$5 | 104.08,42.99 E$2.P$3

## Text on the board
Bottom: S. INVERTER V2I | TN 08/2020
tPlace: In | Gnd | Out
tNames: G | D | S | G | D | S | G | D | S | G | D | S | K | K | AC | AC | FV+ | PE | FV- | K | K | TEPL. | + - | EN. | + - | SITON 210 | SOLAR INVERTER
